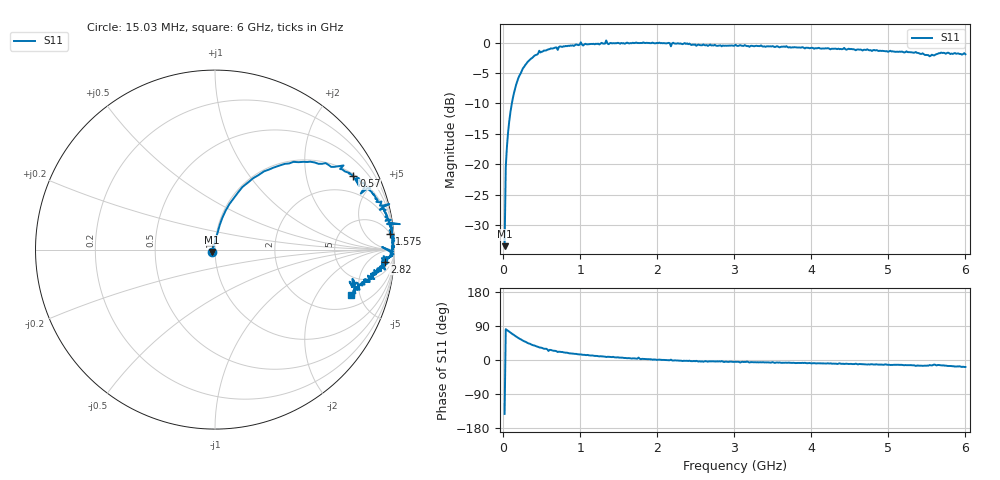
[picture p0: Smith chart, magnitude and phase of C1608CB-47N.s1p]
!	Network	Analyzer	HP8753E.07.74:	Oct	30	2002	Serial	No.	JP38451487
!	Hewlett-Packard
!	7	Sep	2009	9:45:53
!	Frequency	S11
#	HZ	S	RI	R	50
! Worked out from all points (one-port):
!   400 points, 15.03 MHz to 6 GHz, reference 50 ohm
!   lowest |S11| = -33.5 dB at 15.03 MHz (marker M1), VSWR 1.04, Z = 48.3 - j1.26 ohm
!   |S11| at or under -10 dB: start of sweep to 109.4 MHz
!   S11 on the Smith chart (normalised r, x): 15.03 MHz: 0.97, -0.03; 570 MHz: 1.08, +3.72; 1.575 GHz: 5, +21; 2.82 GHz: 14, -18; 6 GHz: 2.95, -4.16
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1.502992e7  -0.0168 -0.013
3.002985e7  0.0143 0.0935
4.502978e7  0.026 0.136
9.002955e7  0.0804 0.254
1.350293e8  0.153 0.349
2.850286e8  0.437 0.489
4.650277e8  0.716 0.469
5.700272e8  0.771 0.409
7.650262e8  0.858 0.333
1.005025e9  0.971 0.254
1.035025e9  0.918 0.222
1.320023e9  0.97 0.15
1.335023e9  1.03 0.142
1.365023e9  0.958 0.143
1.515022e9  0.972 0.106
1.575022e9  0.973 0.0887
1.755021e9  0.984 0.111
1.785021e9  0.991 0.0378
2.145019e9  0.993 -0.0106
2.175019e9  0.931 0.0146
2.265019e9  0.986 -0.0226
2.820016e9  0.945 -0.0673
3.015015e9  0.955 -0.0801
3.765011e9  0.904 -0.116
4.515007e9  0.872 -0.157
5.265004e9  0.81 -0.198
5.595002e9  0.766 -0.163
6e9  0.76 -0.253
